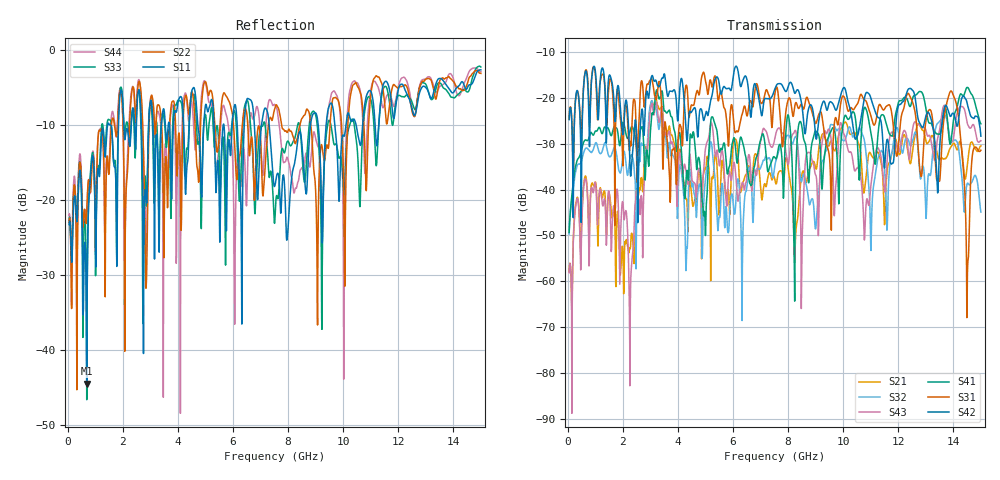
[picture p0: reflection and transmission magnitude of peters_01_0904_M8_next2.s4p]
# MHZ S RI R 50.00
! FREQ  S11  S12  S13  S14
!  S21  S22  S23  S24
!  S31  S32  S33  S34
!  S41  S42  S43  S44
!  REAL  IMAG  REAL  IMAG  REAL  IMAG  REAL  IMAG
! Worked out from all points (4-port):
!   1496 points, 50 MHz to 15 GHz, reference 50 ohm
!   strongest paths, dB at 50 MHz, 3.79 GHz, 7.53 GHz, 11.27 GHz, 15 GHz:
!     S42: -24.7, -18.6, -17.9, -24.3, -28.3
!     S31: -24.6, -31.4, -18.8, -22.2, -31.4
!     S41: -49.3, -24.3, -33.1, -27.6, -25.6
!     S43: -58.2, -29.6, -28.4, -30.9, -29.3
!     S32: -49.7, -32.1, -34.4, -33.1, -44.9
!     S21: -57.9, -28.2, -38.1, -31.9, -30.5
!   lowest |S11| = -44.5 dB at 690 MHz (marker M1), VSWR 1.01, Z = 50.2 + j0.55 ohm
!   |S11| at or under -10 dB: start of sweep to 1.449 GHz; 7.313 GHz to 8.815 GHz (1.502 GHz wide, 18.6 % of centre); 9.695 GHz to 10.1 GHz (406.9 MHz wide, 4.11 % of centre)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
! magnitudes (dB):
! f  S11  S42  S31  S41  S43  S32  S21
! 50 MHz  -23.3  -24.7  -24.6  -49.3  -58.2  -49.7  -57.9
! 690 MHz  -44.5  -14.6  -14.2  -29.3  -39.1  -30.9  -38.5
! 2.28 GHz  -11.9  -37.1  -29.9  -26.8  -61.8  -32.8  -52.4
! 3.05 GHz  -7.3  -15.2  -15.8  -23.7  -21.2  -20.6  -20.6
! 13.93 GHz  -5.7  -23.8  -18.5  -28.8  -29.7  -29.3  -30.5
! 14.52 GHz  -5.0  -21.7  -56.6  -17.7  -25.8  -38.6  -33.9
! 15 GHz  -2.7  -28.3  -31.4  -25.6  -29.3  -44.9  -30.5
